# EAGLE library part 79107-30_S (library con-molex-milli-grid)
RECEPTACAL
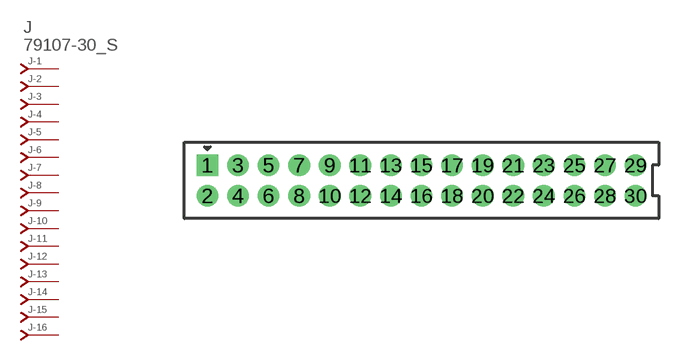
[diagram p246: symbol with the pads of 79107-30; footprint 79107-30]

Designator prefix J; gates -1=J-NV -2=J-N -3=J-N -4=J-N -5=J-N -6=J-N -7=J-N -8=J-N -9=J-N -10=J-N -11=J-N -12=J-N -13=J-N -14=J-N -15=J-N -16=J-N -17=J-N -18=J-N -19=J-N -20=J-N -21=J-N -22=J-N -23=J-N -24=J-N -25=J-N -26=J-N -27=J-N -28=J-N -29=J-N -30=J-N

## 79107-30_S  [79107-30]
1  -1:J  pas
2  -2:J  pas
3  -3:J  pas
4  -4:J  pas
5  -5:J  pas
6  -6:J  pas
7  -7:J  pas
8  -8:J  pas
9  -9:J  pas
10  -10:J  pas
11  -11:J  pas
12  -12:J  pas
13  -13:J  pas
14  -14:J  pas
15  -15:J  pas
16  -16:J  pas
17  -17:J  pas
18  -18:J  pas
19  -19:J  pas
20  -20:J  pas
21  -21:J  pas
22  -22:J  pas
23  -23:J  pas
24  -24:J  pas
25  -25:J  pas
26  -26:J  pas
27  -27:J  pas
28  -28:J  pas
29  -29:J  pas
30  -30:J  pas

## Footprint 79107-30 (pad centres in mm)
RECEPTACAL Dual Row, Vertical, Through-Hole
drill 0.914 square: 1 -14,1
drill 0.914: 2 -14,-1; 3 -12,1; 4 -12,-1; 5 -10,1; 6 -10,-1; 7 -8,1; 8 -8,-1; 9 -6,1; 10 -6,-1; 11 -4,1; 12 -4,-1; 13 -2,1; 14 -2,-1; 15 0,1; 16 0,-1; 17 2,1; 18 2,-1; 19 4,1; 20 4,-1; 21 6,1; 22 6,-1; 23 8,1; 24 8,-1; 25 10,1; 26 10,-1; 27 12,1; 28 12,-1; 29 14,1; 30 14,-1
